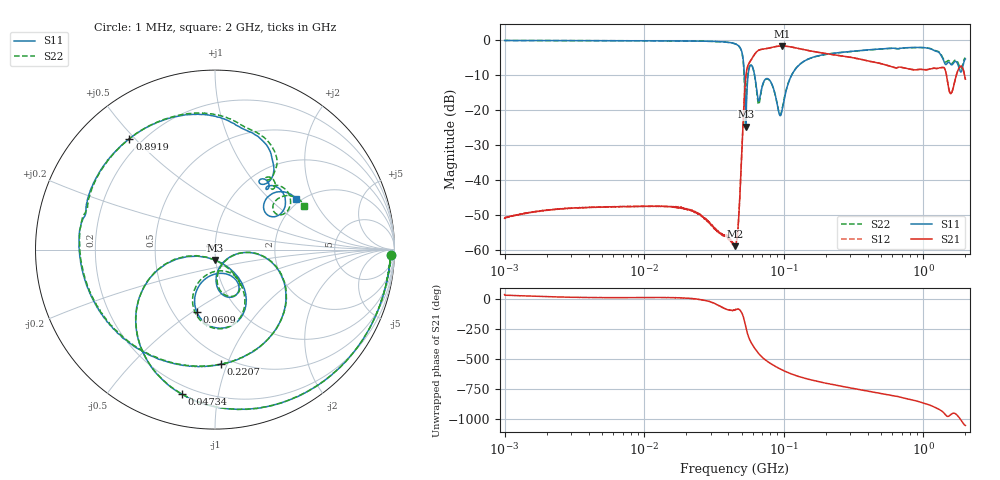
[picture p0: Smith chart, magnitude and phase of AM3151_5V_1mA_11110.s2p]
! Date/Time: Fri Jun 26 11:13:04 2020
! Network Analyzer:  Rev:
! Sweep from 1000000.0 to 2000000000.0, 1601 Points ! Power Supply: 0 V, 0 A
# HZ S DB R 50
!freq MagS11 AngS11 MagS21 AngS21 MagS12 AngS12 MagS22 AngS22
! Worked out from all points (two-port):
!   1601 points, 1 MHz to 2 GHz, reference 50 ohm
!   highest |S21| = -1.72 dB at 97.47 MHz (marker M1); lowest = -58.8 dB at 44.51 MHz (marker M2)
!   |S21| within 3 dB of the highest: 60.39 MHz to 275.2 MHz (214.8 MHz wide, 128 % of centre)
!   lowest |S11| = -24.7 dB at 53.57 MHz (marker M3), VSWR 1.12, Z = 49.8 - j5.81 ohm
!   |S11| at or under -10 dB: 52.16 MHz to 55.53 MHz (3.371 MHz wide, 6.26 % of centre); 61.78 MHz to 114 MHz (52.19 MHz wide, 59.4 % of centre)
!   |S22| runs from -24.6 to -0.2 dB; largest |S21 - S12| = 0.0071
!   S11 on the Smith chart (normalised r, x): 1 MHz: 30, -47; 47.34 MHz: 0.15, -0.79; 60.9 MHz: 0.65, -0.52; 220.7 MHz: 0.44, -0.95; 891.9 MHz: 0.15, +0.48; 2 GHz: 1.88, +1.49
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1000000  -0.17 -1.7  -50.86 39.5  -50.83 35.4  -0.16 -1.7
3555161  -0.20 -5.3  -47.79 15.8  -47.84 15.6  -0.20 -5.3
1.263916e7  -0.27 -18.3  -47.49 14.8  -47.40 14.6  -0.26 -18.2
2.930183e7  -0.40 -45.5  -52.15 -16.7  -52.18 -18.8  -0.40 -45.5
4.450937e7  -1.06 -87.1  -58.80 -91.1  -58.69 -92.9  -1.08 -87.5
4.493426e7  -1.12 -89.1  -58.34 -89.6  -58.40 -89.1  -1.14 -89.6
4.734478e7  -1.65 -102.9  -51.89 -81.6  -51.81 -82.0  -1.69 -103.6
5.036085e7  -3.83 -132.5  -29.47 -121.3  -29.45 -121.3  -4.09 -134.5
5.356903e7  -24.72 -88.6  -10.14 121.3  -10.13 121.3  -20.70 -61.9
5.617532e7  -8.57 -63.4  -6.74 39.1  -6.74 39.1  -8.24 -66.8
6.090023e7  -8.81 -106.3  -4.49 -38.5  -4.49 -38.4  -8.90 -108.7
6.66528e7  -17.23 -73.9  -2.87 -99.9  -2.88 -99.9  -18.10 -71.8
7.57745e7  -11.01 -68.7  -2.44 -158.4  -2.45 -158.4  -11.09 -66.9
9.746975e7  -19.80 -19.3  -1.72 127.3  -1.72 127.2  -19.54 -18.8
1.167534e8  -9.26 -14.9  -2.13 88.2  -2.14 88.3  -9.23 -14.6
1.589914e8  -5.04 -52.9  -3.22 42.4  -3.21 42.4  -5.05 -52.6
2.206635e8  -3.88 -87.1  -4.15 6.5  -4.16 6.5  -3.91 -87.1
5.652395e8  -2.43 -179.7  -7.40 -83.2  -7.37 -83.2  -2.45 178.6
8.918562e8  -2.16 127.7  -8.51 -132.2  -8.50 -132.3  -2.16 125.2
1.413901e9  -6.46 51.7  -8.05 122.7  -8.01 122.7  -5.93 51.8
1.569669e9  -6.94 48.9  -15.31 113.1  -15.35 112.8  -6.51 46.1
2e9  -5.45 32.0  -11.19 22.2  -11.29 21.5  -5.13 25.9
